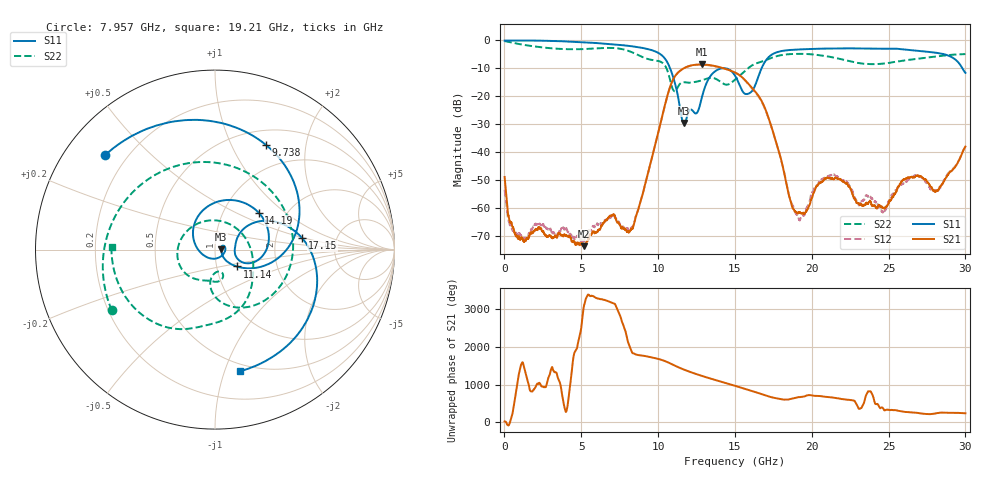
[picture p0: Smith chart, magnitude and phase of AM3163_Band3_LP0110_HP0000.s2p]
!Agilent Technologies,E8364B,MY43040894,A.07.50.67
!Agilent E8364B: A.07.50.67
!Date: Thursday, August 20, 2020 12:13:52
!Correction: S11(Full 2 Port(1,2))
!S21(Full 2 Port(1,2))
!S12(Full 2 Port(1,2))
!S22(Full 2 Port(1,2))
!S2P File: Measurements: S11, S21, S12, S22:
# Hz S  dB  R 50
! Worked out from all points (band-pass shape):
!   3201 points, 10 MHz to 30 GHz, reference 50 ohm
!   highest |S21| = -8.58 dB at 12.85 GHz (marker M1); lowest = -73.5 dB at 5.174 GHz (marker M2)
!   |S21| within 3 dB of the highest: 11.28 GHz to 15.05 GHz (3.774 GHz wide, 28.7 % of centre)
!   lowest |S11| = -29.5 dB at 11.69 GHz (marker M3), VSWR 1.07, Z = 53.5 + j0.124 ohm
!   |S11| at or under -10 dB: 10.78 GHz to 14.11 GHz (3.329 GHz wide, 26.7 % of centre); 14.43 GHz to 16.73 GHz (2.301 GHz wide, 14.8 % of centre); 29.81 GHz to end of sweep
!   |S22| runs from -18.2 to -0.2 dB; largest |S21 - S12| = 0.0069
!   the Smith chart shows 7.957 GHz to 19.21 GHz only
!   S11 on the Smith chart (normalised r, x): 7.957 GHz: 0.12, +0.37; 9.738 GHz: 0.68, +1.37; 11.14 GHz: 1.25, -0.24; 14.19 GHz: 1.46, +0.67; 17.15 GHz: 2.82, +0.48; 19.21 GHz: 0.43, -1.13
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1e7  -0.04 -2.0  -48.80 25.7  -53.37 -8.3  -0.25 -6.5
1.050278e9  -0.00 -28.8  -71.12 46.3  -69.63 74.3  -1.38 -84.7
2.371712e9  -0.08 -65.0  -67.34 -99.9  -66.11 -48.3  -2.43 -168.0
5.014581e9  -0.61 -135.6  -73.10 39.6  -71.00 -127.7  -3.11 51.3
5.173903e9  -0.66 -139.9  -73.53 -147.6  -71.84 -103.9  -3.08 42.4
6.963931e9  -1.32 170.5  -62.65 -61.1  -62.98 -58.2  -2.67 -70.4
7.95735e9  -1.85 139.4  -68.21 103.4  -67.04 126.1  -3.51 -149.5
8.922653e9  -2.60 103.5  -56.26 -28.2  -56.24 -29.1  -5.78 115.2
9.738006e9  -3.76 64.1  -38.92 -90.7  -38.96 -91.9  -7.08 21.6
1.000979e10  -4.43 47.5  -32.90 -117.6  -33.02 -118.8  -7.34 -10.7
1.114379e10  -16.26 -37.7  -12.43 54.0  -12.48 54.1  -17.99 -77.0
1.168736e10  -29.49 2.0  -9.90 -40.9  -9.98 -41.0  -14.92 -88.9
1.284947e10  -20.35 178.4  -8.58 152.3  -8.65 152.3  -14.24 -121.4
1.418965e10  -9.94 40.1  -9.81 -11.6  -9.87 -10.7  -15.28 119.5
1.5005e10  -12.57 -16.3  -11.45 -109.4  -11.43 -109.2  -14.02 0.6
1.715116e10  -6.22 7.6  -27.08 -26.4  -27.31 -24.1  -6.73 -107.4
1.921297e10  -3.21 -78.5  -61.49 -50.3  -64.35 -46.5  -4.78 178.3
2.000958e10  -3.02 -100.1  -56.25 -4.0  -54.70 3.7  -4.97 149.7
2.2868e10  -2.84 -165.8  -57.23 150.2  -57.00 -127.4  -7.91 22.8
2.500479e10  -3.00 144.0  -58.10 -24.3  -57.39 -80.3  -8.05 -87.1
2.73665e10  -3.94 78.3  -49.67 -133.9  -50.28 -128.2  -6.22 -177.8
3e10  -11.57 -28.5  -37.93 -117.3  -38.05 -119.4  -4.87 102.2
